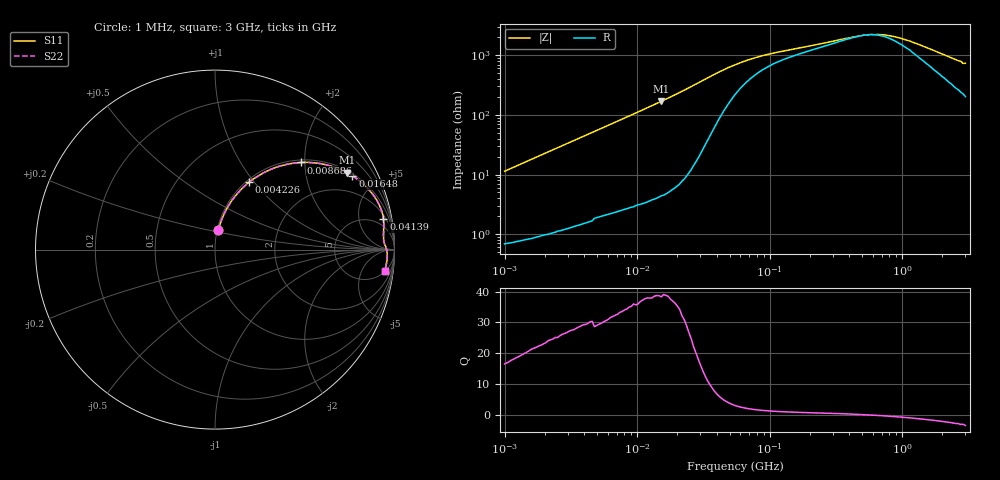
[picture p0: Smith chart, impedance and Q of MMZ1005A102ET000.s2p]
! S-parameter Generated by TDK Corporation
! Copyright(C) 2016 TDK Corporation.
! All Rights Reserved.
! TDK P/N: MMZ1005A102ET000 (Chip Beads)
! Property: |Z|=1000¶ at 100MHz
! Size(LxWxT): 1x0.5x0.5mm, 0.039x0.02x0.02inches
! Model Type: s2p (Touchstone File Format Version 1.0)
! Frequency: DC=Yes Start=1MHz Stop=3000MHz 202points Log-sweep
! Note: This model was converted from impedance.
! Model Generated on May. 16, 2016
! Hash(MD5):
! Port Assignments:
!  1 ---@@@--- 2
! Applicable Conditions:
!  Temperature = 25 degC
!  DC Bias Current = 0 A
!  Small Signal Operation
! Terms and conditions regarding TDK Simulation Models
! (1)This simulation model is being provided solely for informational purposes. Please refer to the specifications of the products in terms of detailed characteristics of such products.
! (2)In no event shall TDK Corporation of any of its subsidiaries be liable for any loss or damage arising, directly or indirectly,
!  From any information contained in this simulation model, including, but not limited to loss or damages arising from any inaccuracies, omissions or errors in connection with such information.
! (3)Any and all copyrights on this simulation model are owned by TDK Corporation.
!  Duplication or redistribution of this simulation model without prior written permission from TDK Corporation is prohibited.
! (4)This simulation model is subject to any modification or change without any prior notice.
! (5)Neither TDK Corporation nor any of its subsidiaries shall make any warranty, express or implied,
!  Including but not limited to the correctness, implied warranties of merchantability and fitness for a particular purpose with respect to this simulation models.
! (6)The use of this simulation model shall be deemed to have consented to the terms and conditions hereof.
# MHz S MA R 50
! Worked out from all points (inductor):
!   201 points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, 1 MHz to 3 GHz, reference 50 ohm
!   read as one part in series: L = 1.8 uH near 1.041 MHz
!   highest Q = 38.7 at 15.21 MHz (marker M1), where L = 1.77 uH
!   self-resonance near 531.5 MHz
!   S11 on the Smith chart (normalised r, x): 1 MHz: 1.01, +0.23; 4.226 MHz: 1.03, +0.94; 8.686 MHz: 1.05, +1.91; 16.48 MHz: 1.09, +3.67; 41.39 MHz: 3, +10; 3 GHz: 5, -14
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1  0.112 80.1  0.987 -6.4  0.987 -6.4  0.112 80.1
2.13957  0.2317 74.2  0.9632 -13.4  0.9632 -13.4  0.2317 74.2
3.900413  0.3933 64.9  0.906 -23.1  0.906 -23.1  0.3933 64.9
4.225536  0.4195 63.3  0.8937 -24.8  0.8937 -24.8  0.4195 63.3
6.305767  0.5631 53.9  0.8087 -34.3  0.8087 -34.3  0.5631 53.9
8.686058  0.6815 45.4  0.7125 -42.9  0.7125 -42.9  0.6815 45.4
11.04425  0.7626 38.8  0.6267 -49.7  0.6267 -49.7  0.7626 38.8
14.61624  0.8412 31.3  0.5195 -57.2  0.5195 -57.2  0.8412 31.3
15.21322  0.8507 30.2  0.5039 -58.3  0.5039 -58.3  0.8507 30.2
16.48134  0.8689 28.2  0.4731 -60.3  0.4731 -60.3  0.8689 28.2
25.59965  0.9369 18.3  0.3137 -69.4  0.3137 -69.4  0.9369 18.3
41.38676  0.954 10.4  0.1827 -70.3  0.1827 -70.3  0.954 10.4
54.77226  0.9482 7.5  0.137 -64.1  0.137 -64.1  0.9482 7.5
88.54986  0.9416 4.5  0.09544 -50.1  0.09544 -50.1  0.9416 4.5
213.6344  0.9449 1.9  0.06419 -29.9  0.06419 -29.9  0.9449 1.9
515.4121  0.9562 0.1  0.04387 -2.2  0.04387 -2.2  0.9562 0.1
655.3423  0.9581 -0.5  0.04292 12.0  0.04292 12.0  0.9581 -0.5
800.5644  0.9592 -1.1  0.04505 24.4  0.04505 24.4  0.9592 -1.1
1147.801  0.9601 -2.3  0.05561 43.1  0.05561 43.1  0.9601 -2.3
2769.173  0.9569 -6.6  0.1204 65.8  0.1204 65.8  0.9569 -6.6
2882.277  0.952 -7.1  0.1306 64.9  0.1306 64.9  0.952 -7.1
3000  0.9562 -7.2  0.1301 66.8  0.1301 66.8  0.9562 -7.2
